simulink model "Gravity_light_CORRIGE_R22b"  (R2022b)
settings: Solver=VariableStepAuto  StartTime=0.0  StopTime=20*60  RelTol=1e-3
libraries: fl_lib x19, nesl_utility x5

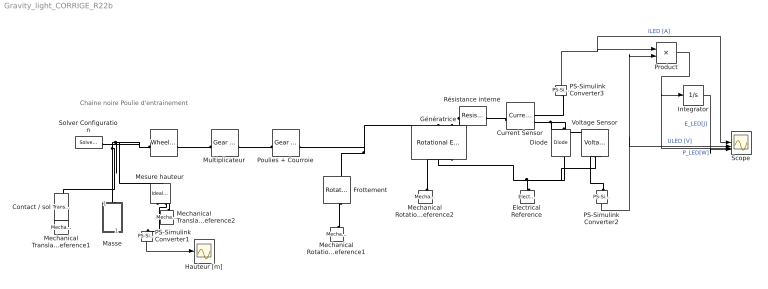
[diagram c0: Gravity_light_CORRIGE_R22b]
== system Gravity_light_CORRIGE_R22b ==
  note: Chaine noire Poulie d'entrainement
  " " : fl_lib/Mechanical/Mechanisms/Wheel and Axle  R=11 mm  or=1  t_specify=off  t_priority=None  t=0 N*m  t_nominal_specify=off  t_nominal_unit=N*m  t_nominal_value=1  f_specify=off  f_priority=None  f=0 N  f_nominal_specify=off  f_nominal_unit=N  f_nominal_value=1
  Contact / sol : fl_lib/Mechanical/Translational Elements/Translational Hard Stop  upper_bnd=2 m  lower_bnd=0 m  stiff_up=1e6 N/m  stiff_low=1e6 N/m  D_up=150 N/(m/s)  D_low=150 N/(m/s)  model=1  transition=0.1 mm  v_specify=off  v_priority=None  v=0 m/s  v_nominal_specify=off  v_nominal_unit=m/s  v_nominal_value=1  f_specify=off  f_priority=None  f=0 N  f_nominal_specify=off  f_nominal_unit=N  f_nominal_value=1  x_specify=off  x_priority=High  x=0 m  x_nominal_specify=off  x_nominal_unit=m  x_nominal_value=1
  Current Sensor : fl_lib/Electrical/Electrical Sensors/Current Sensor
  Diode : fl_lib/Electrical/Electrical Elements/Diode  Vf=2.55 V  Ron=2.5 Ohm  Goff=1e-8 1/Ohm  i_specify=off  i_priority=None  i=0 A  i_nominal_specify=off  i_nominal_unit=A  i_nominal_value=1  v_specify=off  v_priority=None  v=0 V  v_nominal_specify=off  v_nominal_unit=V  v_nominal_value=1
  Electrical Reference : fl_lib/Electrical/Electrical Elements/Electrical Reference
  Frottement : fl_lib/Mechanical/Rotational Elements/Rotational Friction  brkwy_trq=0.000290 N*m  brkwy_vel=0.00000017 rad/s  Col_trq=0.000290 N*m  visc_coef=0.00000017 N*m/(rad/s)  w_specify=off  w_priority=None  w=0 rad/s  w_nominal_specify=off  w_nominal_unit=rad/s  w_nominal_value=1  t_specify=off  t_priority=None  t=0 N*m  t_nominal_specify=off  t_nominal_unit=N*m  t_nominal_value=1
  Génératrice : fl_lib/Electrical/Electrical Elements/Rotational Electromechanical Converter  K=0.0206 V/(rad/s)  i_specify=off  i_priority=None  i=0 A  i_nominal_specify=off  i_nominal_unit=A  i_nominal_value=1  v_specify=off  v_priority=None  v=0 V  v_nominal_specify=off  v_nominal_unit=V  v_nominal_value=1  t_specify=off  t_priority=None  t=0 N*m  t_nominal_specify=off  t_nominal_unit=N*m  t_nominal_value=1  w_specify=off  w_priority=None  w=0 rad/s  w_nominal_specify=off  w_nominal_unit=rad/s  w_nominal_value=1
  Hauteur [m] : Scope
  Integrator : Integrator
  Masse : Subsystem  mask(Masse et son Poids){m=12}
      mask prompts: m "Masse [kg]"
      mask help: Masse dans un champ de pesanteur
  Mechanical Rotational Reference1 : fl_lib/Mechanical/Rotational Elements/Mechanical Rotational Reference
  Mechanical Rotational Reference2 : fl_lib/Mechanical/Rotational Elements/Mechanical Rotational Reference
  Mechanical Translational Reference1 : fl_lib/Mechanical/Translational Elements/Mechanical Translational Reference
  Mechanical Translational Reference2 : fl_lib/Mechanical/Translational Elements/Mechanical Translational Reference
  Mesure hauteur : fl_lib/Mechanical/Mechanical Sensors/Ideal Translational Motion Sensor  reference=foundation.enum.MeasurementReference.difference  acceleration_port=false  velocity_port=true  position_port=true  offset=0 m
  Multiplicateur : fl_lib/Mechanical/Mechanisms/Gear Box  ratio=140*2  t_in_specify=off  t_in_priority=None  t_in=0 N*m  t_in_nominal_specify=off  t_in_nominal_unit=N*m  t_in_nominal_value=1  t_out_specify=off  t_out_priority=None  t_out=0 N*m  t_out_nominal_specify=off  t_out_nominal_unit=N*m  t_out_nominal_value=1
  PS-Simulink Converter1 : nesl_utility/PS-Simulink Converter  PhysicalDomain=network_engine_domain  SubClassName=ps_output  LeftPortType=input  RightPortType=output  PseudoPeriodic=off  Frequencies=[]  VectorFormat=1-D array  Unit=1  AffineConversion=off
  PS-Simulink Converter2 : nesl_utility/PS-Simulink Converter  PhysicalDomain=network_engine_domain  SubClassName=ps_output  LeftPortType=input  RightPortType=output  PseudoPeriodic=off  Frequencies=[]  VectorFormat=1-D array  Unit=1  AffineConversion=off
  PS-Simulink Converter3 : nesl_utility/PS-Simulink Converter  PhysicalDomain=network_engine_domain  SubClassName=ps_output  LeftPortType=input  RightPortType=output  PseudoPeriodic=off  Frequencies=[]  VectorFormat=1-D array  Unit=1  AffineConversion=off
  Poulies + Courroie : fl_lib/Mechanical/Mechanisms/Gear Box  ratio=60/12  t_in_specify=off  t_in_priority=None  t_in=0 N*m  t_in_nominal_specify=off  t_in_nominal_unit=N*m  t_in_nominal_value=1  t_out_specify=off  t_out_priority=None  t_out=0 N*m  t_out_nominal_specify=off  t_out_nominal_unit=N*m  t_out_nominal_value=1
  Product : Product
  Résistance interne : fl_lib/Electrical/Electrical Elements/Resistor  R=21.5 Ohm  i_specify=off  i_priority=None  i=0 A  i_nominal_specify=off  i_nominal_unit=A  i_nominal_value=1  v_specify=off  v_priority=None  v=0 V  v_nominal_specify=off  v_nominal_unit=V  v_nominal_value=1
  Scope : Scope  NumInputPorts=4
  Solver Configuration : nesl_utility/Solver Configuration  PhysicalDomain=network_engine_domain  SubClassName=solver  LeftPortType=input  RightPortType=generic  Tones=[]  Harmonics=[]  SimulateNoise=off  Profile=off  UseLocalSampling=off  EnableSwitchedLinearOptims=on  FrequencyDomain=off  UseCCode=off  RelTol=0.001  AbsTol=1e-06  MinStep=1e-09  ToWorkspace=off  RevertToSquareIcSolve=off  NumHomotopyIterations=100  PhasorMode=off  PhasorModeNumHarmonics=1  ConsistencySolver=NEWTON_FTOL  IndexReductionMethod=DerivativeReplacement  DoDC=off  ResidualTolerance=1e-09  ConsistencyTolSource=GLOBAL  ConsistencyAbsTol=0.001  ConsistencyRelTol=0.001  ConsistencyTolFactor=0.001  UseLocalSolver=off  LocalSolverChoice=NE_BACKWARD_EULER_ADVANCER  ResolveIndetEquations=on  FunctionEvalNumThread=1  LocalSolverSampleTime=0.001  DoFixedCost=off  MaxNonlinIter=3  MaxModeIter=2  ComputeImpulses=off  ImpulseIterations=2  LinearAlgebra=auto  LinearAlgebraNumThread=0  EquationFormulation=NE_TIME_EF  DelaysMemoryBudget=1024  AutomaticFiltering=on  FilteringTimeConstant=0.001  PartitionStorageMethod=AS_NEEDED  PartitionMemoryBudget=1024  PartitionMethod=FAST
  Voltage Sensor : fl_lib/Electrical/Electrical Sensors/Voltage Sensor
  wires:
  PS-Simulink Converter3/1 -> Product/1, Scope/1  "ILED [A]"
  PS-Simulink Converter2/1 -> Product/2, Scope/2  "ULED [V]"
  PS-Simulink Converter1/1 -> Hauteur [m]/1
  Product/1 -> Integrator/1, Scope/3  "P_LED[W]"
  Integrator/1 -> Scope/4  "E_LED[J]"
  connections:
  " "/RConn1 -- Solver Configuration/RConn1 -- Mesure hauteur/LConn1 -- Masse/LConn1 -- Contact / sol/LConn1
  Mechanical Translational Reference2/LConn1 -- Mesure hauteur/RConn1
  Mechanical Translational Reference1/LConn1 -- Contact / sol/RConn1
  Electrical Reference/LConn1 -- Voltage Sensor/RConn2 -- Diode/RConn1 -- Génératrice/RConn1
  Génératrice/LConn2 -- Frottement/LConn1 -- Poulies + Courroie/LConn1
  Résistance interne/RConn1 -- Génératrice/LConn1
  Mechanical Rotational Reference2/LConn1 -- Génératrice/RConn2
  Current Sensor/LConn1 -- Résistance interne/LConn1
  Current Sensor/RConn2 -- Voltage Sensor/LConn1 -- Diode/LConn1
  Mesure hauteur/RConn3 -- PS-Simulink Converter1/LConn1
  PS-Simulink Converter3/LConn1 -- Current Sensor/RConn1
  PS-Simulink Converter2/LConn1 -- Voltage Sensor/RConn1
  " "/LConn1 -- Multiplicateur/RConn1
  Multiplicateur/LConn1 -- Poulies + Courroie/RConn1
  Mechanical Rotational Reference1/LConn1 -- Frottement/RConn1

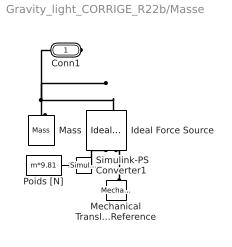
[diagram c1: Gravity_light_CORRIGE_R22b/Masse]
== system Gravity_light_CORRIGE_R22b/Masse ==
  Ideal Force Source : fl_lib/Mechanical/Mechanical Sources/Ideal Force Source
  Mass : fl_lib/Mechanical/Translational Elements/Mass  mass=m kg  num_ports=foundation.enum.numPorts2.one  v_specify=off  v_priority=High  v=0 m/s  v_nominal_specify=off  v_nominal_unit=m/s  v_nominal_value=1  f_specify=off  f_priority=None  f=0 N  f_nominal_specify=off  f_nominal_unit=N  f_nominal_value=1
  Mechanical Translational Reference : fl_lib/Mechanical/Translational Elements/Mechanical Translational Reference
  Poids [N] : Constant  Value=m*9.81
  Simulink-PS Converter1 : nesl_utility/Simulink-PS Converter  PhysicalDomain=network_engine_domain  SubClassName=ps_input  LeftPortType=input  RightPortType=output  PseudoPeriodic=off  Frequencies=[]  NoiseDistribution=none  NoiseParameters=[]  Unit=1  AffineConversion=off  FilteringAndDerivatives=provide  SimscapeFilterOrder=1  InputFilterTimeConstant=0.001  UdotUserProvided=0
  Conn1 : PMIOPort  Side=Left
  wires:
  Poids [N]/1 -> Simulink-PS Converter1/1
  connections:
  Mechanical Translational Reference/LConn1 -- Ideal Force Source/RConn2
  Mass/LConn1 -- Conn1/RConn1 -- Ideal Force Source/LConn1
  Simulink-PS Converter1/RConn1 -- Ideal Force Source/RConn1
